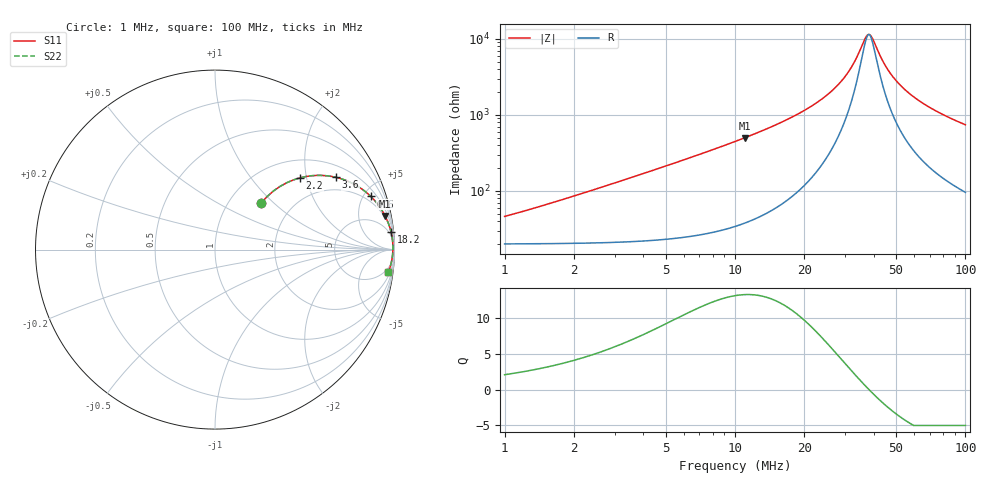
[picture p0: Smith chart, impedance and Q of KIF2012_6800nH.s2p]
!version-2
!date-12.2020
!Series
# MHz S RI R 50
!Freq ReS11 ImS11 ReS21 ImS21 ReS12 ImS12 ReS22 ImS22
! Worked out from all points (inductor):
!   496 points, 1 MHz to 100 MHz, reference 50 ohm
!   read as one part in series: L = 6.59 uH near 1.6 MHz
!   highest Q = 13.2 at 11 MHz (marker M1), where L = 7.18 uH
!   self-resonance near 38.15 MHz
!   S11 on the Smith chart (normalised r, x): 1 MHz: 1.40, +0.83; 2.2 MHz: 1.41, +1.83; 3.6 MHz: 1.43, +3.01; 6.6 MHz: 1.51, +5.63; 18.2 MHz: 3, +19; 100 MHz: 3, -15
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1  0.2553 0.2569  0.7447 -0.2569  0.7447 -0.2569  0.2553 0.2569
2.2  0.4729 0.3997  0.5271 -0.3997  0.5271 -0.3997  0.4729 0.3997
3.6  0.6747 0.4025  0.3253 -0.4025  0.3253 -0.4025  0.6747 0.4025
5  0.7931 0.3542  0.2069 -0.3542  0.2069 -0.3542  0.7931 0.3542
6.6  0.8679 0.2964  0.1321 -0.2964  0.1321 -0.2964  0.8679 0.2964
11  0.9482 0.1871  0.0518 -0.1871  0.0518 -0.1871  0.9482 0.1871
17.6  0.9793 0.1042  0.0207 -0.1042  0.0207 -0.1042  0.9793 0.1042
18.2  0.9806 0.099  0.0194 -0.099  0.0194 -0.099  0.9806 0.099
28  0.9903 0.0387  0.00974 -0.0387  0.00974 -0.0387  0.9903 0.0387
31.2  0.9911 0.0249  0.0089 -0.0249  0.0089 -0.0249  0.9911 0.0249
34  0.9914 0.0142  0.0086 -0.0142  0.0086 -0.0142  0.9914 0.0142
36.8  0.9914 0.00442  0.0086 -0.00442  0.0086 -0.00442  0.9914 0.00442
37.6  0.9914 0.00177  0.00865 -0.00177  0.00865 -0.00177  0.9914 0.00177
38.4  0.9913 -0.000814  0.00871 0.000814  0.00871 0.000814  0.9913 -0.000814
39.4  0.9912 -0.00397  0.00881 0.00397  0.00881 0.00397  0.9912 -0.00397
42.6  0.9907 -0.0135  0.00928 0.0135  0.00928 0.0135  0.9907 -0.0135
44.8  0.9903 -0.0197  0.00973 0.0197  0.00973 0.0197  0.9903 -0.0197
50.6  0.9888 -0.0347  0.0112 0.0347  0.0112 0.0347  0.9888 -0.0347
57.6  0.9864 -0.051  0.0136 0.051  0.0136 0.051  0.9864 -0.051
67  0.9826 -0.0706  0.0174 0.0706  0.0174 0.0706  0.9826 -0.0706
83.6  0.9748 -0.1009  0.0252 0.1009  0.0252 0.1009  0.9748 -0.1009
100  0.9661 -0.1273  0.0339 0.1273  0.0339 0.1273  0.9661 -0.1273
